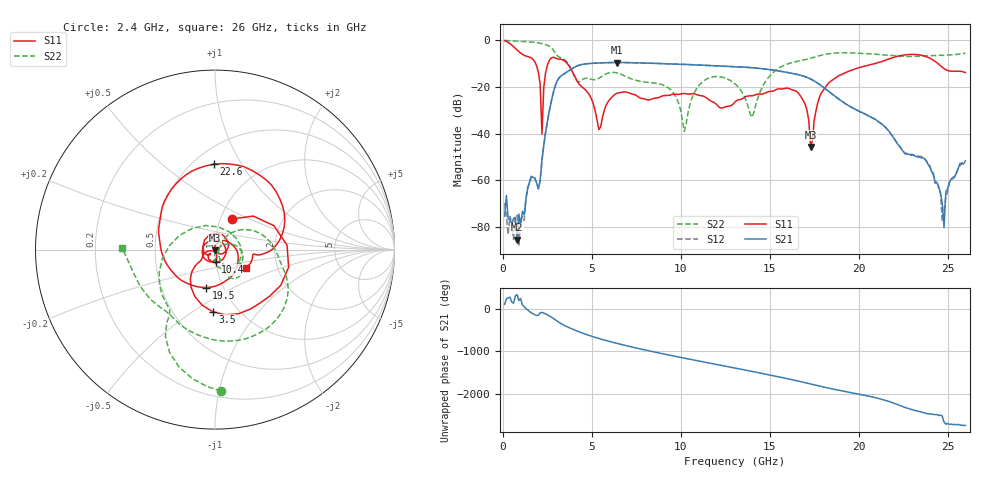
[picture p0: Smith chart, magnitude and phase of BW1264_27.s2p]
!Keysight Technologies,N5245B,MY57181159,A.13.60.06
!Date: Friday, December 18, 2020 23:53:21
!Correction: S11(Full 2 Port(1,2))
!S21(Full 2 Port(1,2))
!S12(Full 2 Port(1,2))
!S22(Full 2 Port(1,2))
!S2P File: Measurements: S11, S21, S12, S22:
# Hz S  dB  R 50
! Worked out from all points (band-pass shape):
!   260 points, 100 MHz to 26 GHz, reference 50 ohm
!   highest |S21| = -9.71 dB at 6.4 GHz (marker M1); lowest = -85.3 dB at 800 MHz (marker M2)
!   |S21| within 3 dB of the highest: 3.811 GHz to 14.96 GHz (11.15 GHz wide, 119 % of centre)
!   lowest |S11| = -45.8 dB at 17.3 GHz (marker M3), VSWR 1.01, Z = 50.2 - j0.482 ohm
!   |S11| at or under -10 dB: 1.833 GHz to 2.549 GHz (715.6 MHz wide, 32.7 % of centre); 3.603 GHz to 20.98 GHz (17.38 GHz wide, 141 % of centre); 24.43 GHz to end of sweep
!   |S22| runs from -39.1 to -0.3 dB; largest |S21 - S12| = 0.00061
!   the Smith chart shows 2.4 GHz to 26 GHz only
!   S11 on the Smith chart (normalised r, x): 2.4 GHz: 1.13, +0.40; 3.5 GHz: 0.77, -0.60; 10.4 GHz: 1.00, -0.14; 19.5 GHz: 0.83, -0.37; 22.6 GHz: 0.62, +0.77; 26 GHz: 1.37, -0.30
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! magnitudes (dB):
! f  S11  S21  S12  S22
! 100 MHz  -0.4  -75.2  -69.7  -0.3
! 800 MHz  -4.3  -85.3  -74.9  -0.6
! 1.9 GHz  -11.1  -61.0  -61.2  -1.2
! 2.2 GHz  -40.2  -51.4  -51.2  -1.6
! 2.4 GHz  -14.2  -39.7  -39.8  -2.1
! 3.5 GHz  -9.2  -14.3  -14.3  -8.7
! 4.5 GHz  -20.4  -10.5  -10.5  -16.9
! 5.4 GHz  -38.3  -9.9  -9.9  -16.4
! 6.4 GHz  -22.9  -9.7  -9.7  -14.1
! 8.8 GHz  -24.5  -10.1  -10.1  -18.9
! 10.4 GHz  -23.2  -10.6  -10.6  -31.5
! 13.1 GHz  -26.2  -11.5  -11.5  -19.1
! 14 GHz  -23.9  -11.9  -11.9  -33.1
! 16.5 GHz  -22.0  -14.7  -14.7  -9.3
! 17.3 GHz  -45.8  -16.7  -16.8  -7.9
! 17.4 GHz  -43.0  -17.1  -17.1  -7.7
! 19.5 GHz  -13.3  -28.4  -28.3  -5.6
! 21.7 GHz  -8.2  -39.0  -38.9  -6.6
! 22.6 GHz  -6.5  -48.6  -48.5  -7.1
! 24.2 GHz  -8.7  -56.9  -57.9  -6.8
! 24.8 GHz  -12.3  -80.2  -72.8  -6.6
! 26 GHz  -14.0  -51.6  -52.3  -5.7
